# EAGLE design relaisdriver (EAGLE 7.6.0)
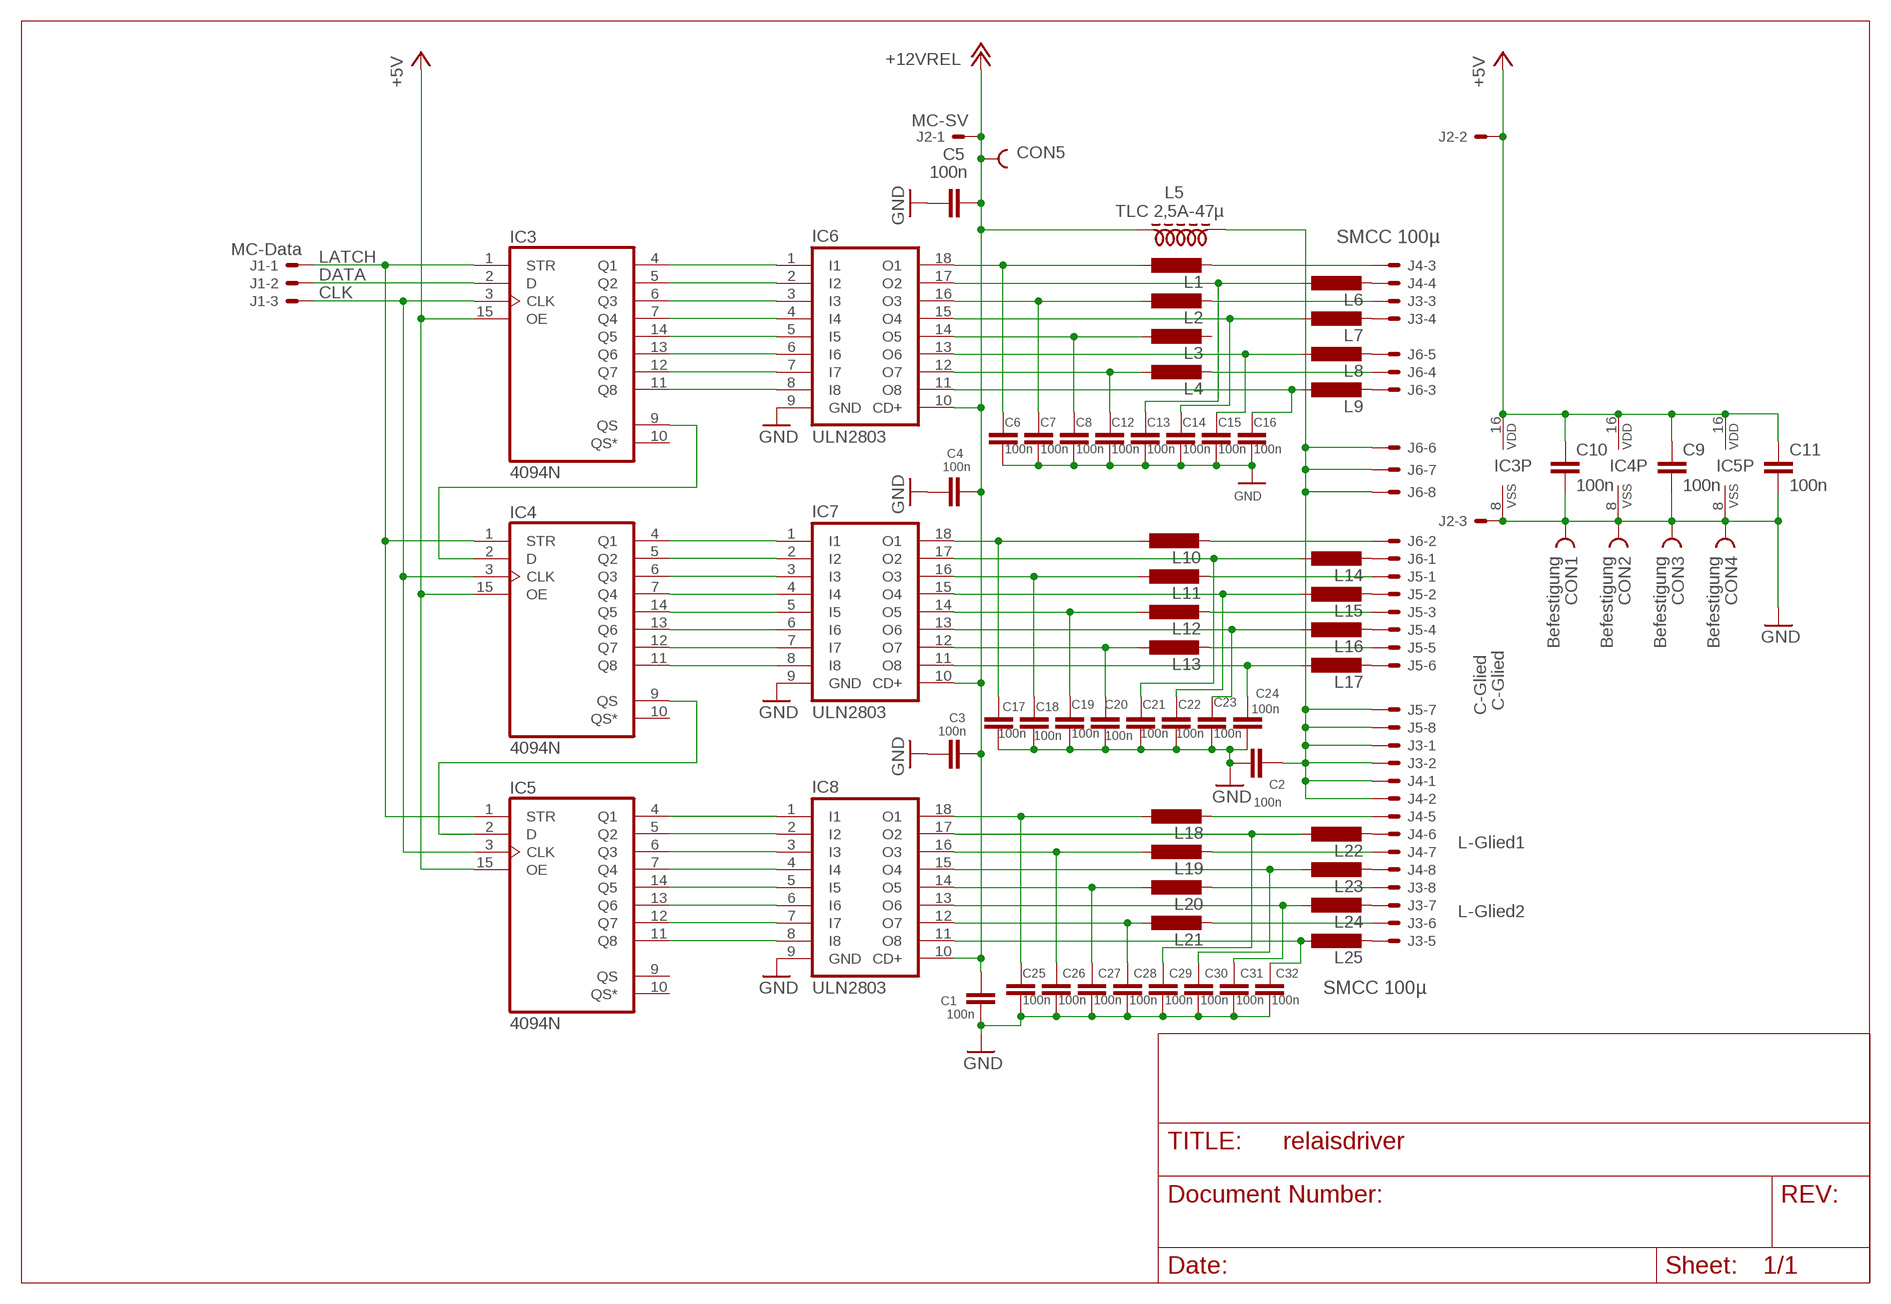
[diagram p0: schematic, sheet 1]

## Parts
C1  100n  C-EUC0805  [C0805]
C2  100n  C-EUC0805  [C0805]
C3  100n  C-EUC0805  [C0805]
C4  100n  C-EUC0805  [C0805]
C5  100n  C-EUC0805  [C0805]
C6  100n  C-EUC0805  [C0805]
C7  100n  C-EUC0805  [C0805]
C8  100n  C-EUC0805  [C0805]
C9  100n  C-EUC0805  [C0805]
C10  100n  C-EUC0805  [C0805]
C11  100n  C-EUC0805  [C0805]
C12  100n  C-EUC0805  [C0805]
C13  100n  C-EUC0805  [C0805]
C14  100n  C-EUC0805  [C0805]
C15  100n  C-EUC0805  [C0805]
C16  100n  C-EUC0805  [C0805]
C17  100n  C-EUC0805  [C0805]
C18  100n  C-EUC0805  [C0805]
C19  100n  C-EUC0805  [C0805]
C20  100n  C-EUC0805  [C0805]
C21  100n  C-EUC0805  [C0805]
C22  100n  C-EUC0805  [C0805]
C23  100n  C-EUC0805  [C0805]
C24  100n  C-EUC0805  [C0805]
C25  100n  C-EUC0805  [C0805]
C26  100n  C-EUC0805  [C0805]
C27  100n  C-EUC0805  [C0805]
C28  100n  C-EUC0805  [C0805]
C29  100n  C-EUC0805  [C0805]
C30  100n  C-EUC0805  [C0805]
C31  100n  C-EUC0805  [C0805]
C32  100n  C-EUC0805  [C0805]
CON1  Befestigung  PIN2_53MM  [HOLE3]
CON2  Befestigung  PIN2_53MM  [HOLE3]
CON3  Befestigung  PIN2_53MM  [HOLE3]
CON4  Befestigung  PIN2_53MM  [HOLE3]
CON5  PIN1_75OV  [PIN_1,75OV]
IC3  4094N  [DIL16]
IC4  4094N  [DIL16]
IC5  4094N  [DIL16]
IC6  ULN2803  ULN2803A  [DIL18]
IC7  ULN2803  ULN2803A  [DIL18]
IC8  ULN2803  ULN2803A  [DIL18]
J1  MC-Data  22-27-2031-03  [6410-03]
J2  MC-SV  22-27-2031-03  [6410-03]
J3  L-Glied2  22-27-2081-08  [6410-08]
J4  L-Glied1  22-27-2081-08  [6410-08]
J5  C-Glied  22-27-2081-08  [6410-08]
J6  C-Glied  22-27-2081-08  [6410-08]
L1  L-EU0207/10  [0207/10]
L2  L-EU0207/10  [0207/10]
L3  L-EU0207/10  [0207/10]
L4  L-EU0207/10  [0207/10]
L5  TLC 2,5A-47µ  Z28/70CW  [Z28/7]
L6  L-EU0207/10  [0207/10]
L7  L-EU0207/10  [0207/10]
L8  L-EU0207/10  [0207/10]
L9  L-EU0207/10  [0207/10]
L10  L-EU0207/10  [0207/10]
L11  L-EU0207/10  [0207/10]
L12  L-EU0207/10  [0207/10]
L13  L-EU0207/10  [0207/10]
L14  L-EU0207/10  [0207/10]
L15  L-EU0207/10  [0207/10]
L16  L-EU0207/10  [0207/10]
L17  L-EU0207/10  [0207/10]
L18  L-EU0207/10  [0207/10]
L19  L-EU0207/10  [0207/10]
L20  L-EU0207/10  [0207/10]
L21  L-EU0207/10  [0207/10]
L22  L-EU0207/10  [0207/10]
L23  L-EU0207/10  [0207/10]
L24  L-EU0207/10  [0207/10]
L25  L-EU0207/10  [0207/10]

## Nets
+5V: C9.1 C10.1 C11.1 IC3.15(OE) IC3.16(VDD) IC4.15(OE) IC4.16(VDD) IC5.15(OE) IC5.16(VDD) J2.2
+12VREL: C1.1 C3.1 C4.1 C5.1 CON5.1 IC6.10(CD+) IC7.10(CD+) IC8.10(CD+) J2.1 L5.1 ; supply symbol labelled +12V
CLK: IC3.3(CLK) IC4.3(CLK) IC5.3(CLK) J1.3
DATA: IC3.2(D) J1.2
GND: C1.2 C2.2 C3.2 C4.2 C5.2 C6.2 C7.2 C8.2 C9.2 C10.2 C11.2 C12.2 C13.2 C14.2 C15.2 C16.2 C17.2 C18.2 C19.2 C20.2 C21.2 C22.2 C23.2 C24.2 C25.2 C26.2 C27.2 C28.2 C29.2 C30.2 C31.2 C32.2 CON1.1 CON2.1 CON3.1 CON4.1 IC3.8(VSS) IC4.8(VSS) IC5.8(VSS) IC6.9(GND) IC7.9(GND) IC8.9(GND) J2.3
LATCH: IC3.1(STR) IC4.1(STR) IC5.1(STR) J1.1
N$1: C6.1 IC6.18(O1) L1.1
N$2: C7.1 IC6.16(O3) L2.1
N$3: IC4.7(Q4) IC7.4(I4)
N$4: IC4.14(Q5) IC7.5(I5)
N$5: IC4.13(Q6) IC7.6(I6)
N$6: C8.1 IC6.14(O5) L3.1
N$7: C12.1 IC6.12(O7) L4.1
N$8: C16.1 IC6.11(O8) L9.1
N$9: IC3.4(Q1) IC6.1(I1)
N$10: C15.1 IC6.13(O6) L8.1
N$11: C14.1 IC6.15(O4) L7.1
N$12: IC4.12(Q7) IC7.7(I7)
N$13: C13.1 IC6.17(O2) L6.1
N$14: IC4.11(Q8) IC7.8(I8)
N$15: J4.4 L6.2
N$16: J3.5 L25.2
N$17: J3.6 L21.2
N$18: J6.4 L4.2
N$19: J6.2 L10.2
N$20: J5.1 L11.2
N$21: IC3.5(Q2) IC6.2(I2)
N$22: IC3.6(Q3) IC6.3(I3)
N$23: IC3.9(QS) IC4.2(D)
N$24: IC4.9(QS) IC5.2(D)
N$25: IC3.7(Q4) IC6.4(I4)
N$26: IC3.14(Q5) IC6.5(I5)
N$27: IC3.13(Q6) IC6.6(I6)
N$28: IC3.12(Q7) IC6.7(I7)
N$29: IC3.11(Q8) IC6.8(I8)
N$30: IC4.4(Q1) IC7.1(I1)
N$31: IC4.5(Q2) IC7.2(I2)
N$32: IC4.6(Q3) IC7.3(I3)
N$33: J5.3 L12.2
N$34: J5.5 L13.2
N$35: J4.8 L23.2
N$36: C17.1 IC7.18(O1) L10.1
N$37: C18.1 IC7.16(O3) L11.1
N$38: IC5.4(Q1) IC8.1(I1)
N$39: IC5.5(Q2) IC8.2(I2)
N$40: IC5.6(Q3) IC8.3(I3)
N$41: IC5.7(Q4) IC8.4(I4)
N$42: IC5.14(Q5) IC8.5(I5)
N$43: IC5.13(Q6) IC8.6(I6)
N$44: IC5.12(Q7) IC8.7(I7)
N$45: IC5.11(Q8) IC8.8(I8)
N$46: C19.1 IC7.14(O5) L12.1
N$47: C20.1 IC7.12(O7) L13.1
N$48: C24.1 IC7.11(O8) L17.1
N$49: C23.1 IC7.13(O6) L16.1
N$50: C22.1 IC7.15(O4) L15.1
N$51: C21.1 IC7.17(O2) L14.1
N$52: C2.1 J3.1 J3.2 J4.1 J4.2 J5.7 J5.8 J6.6 J6.7 J6.8 L5.2
N$53: J5.6 L17.2
N$54: J5.4 L16.2
N$55: J5.2 L15.2
N$56: J6.1 L14.2
N$57: J6.3 L9.2
N$58: J6.5 L8.2
N$59: J3.7 L24.2
N$60: C25.1 IC8.18(O1) L18.1
N$61: C26.1 IC8.16(O3) L19.1
N$62: C27.1 IC8.14(O5) L20.1
N$63: C28.1 IC8.12(O7) L21.1
N$64: C32.1 IC8.11(O8) L25.1
N$65: C31.1 IC8.13(O6) L24.1
N$66: C30.1 IC8.15(O4) L23.1
N$67: C29.1 IC8.17(O2) L22.1
N$68: J4.5 L18.2
N$69: J4.6 L22.2
N$70: J4.7 L19.2
N$71: J4.3 L1.2
N$72: J3.8 L20.2
N$73: J3.4 L7.2
N$74: J3.3 L2.2
Unconnected: IC3.10(QS*) IC4.10(QS*) IC5.9(QS) IC5.10(QS*) L3.2

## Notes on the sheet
- SMCC 100µ
- SMCC 100µ

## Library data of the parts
C1-C32 = rcl:C-EU: CAPACITOR, European symbol
CON1-CON4 = lindenau:PIN2_5
CON5 = lindenau:PIN1_75
IC3-IC5 = 40xx:4094: 8-stage SHIFT/STORE REGISTER, tri-state
IC6-IC8 = uln-udn:ULN2803A: DRIVER ARRAY
J1 J2 = con-molex:22-?-03: CONNECTOR wire to board 2.54 mm (.1 inch) pitch header; OC_FARNELL: unknown; OC_NEWARK: unknown
J3-J6 = con-molex:22-?-08: CONNECTOR wire to board 2.54 mm (.1 inch) pitch header; OC_FARNELL: unknown; OC_NEWARK: unknown
L1-L4 L6-L25 = rcl:L-EU: INDUCTOR, European symbol
L5 = inductor-neosid:Z?CW: CHOKE; OC_FARNELL: unknown; OC_NEWARK: unknown

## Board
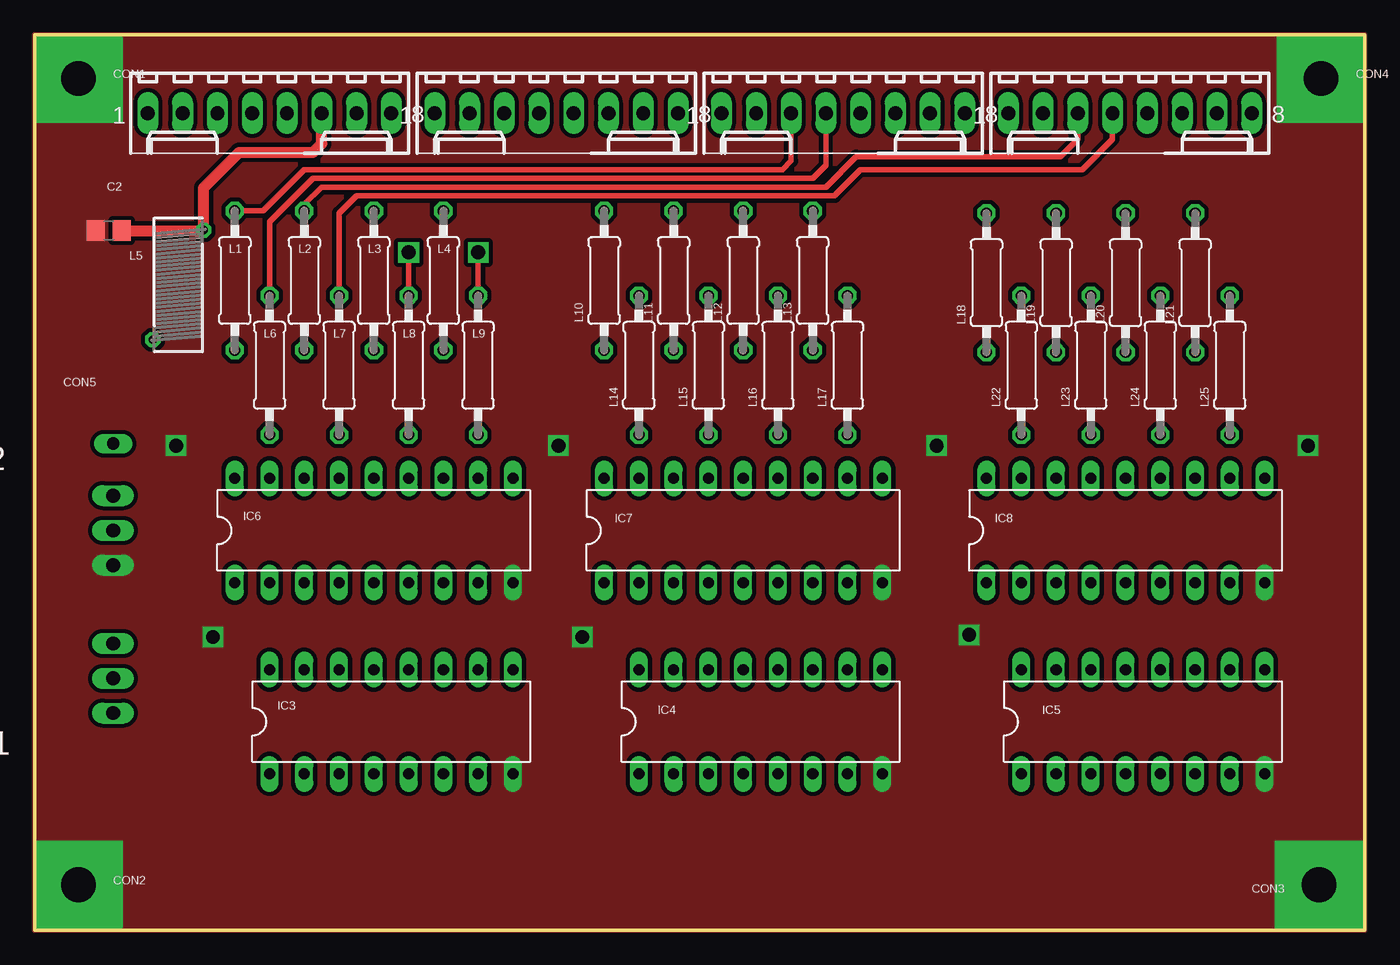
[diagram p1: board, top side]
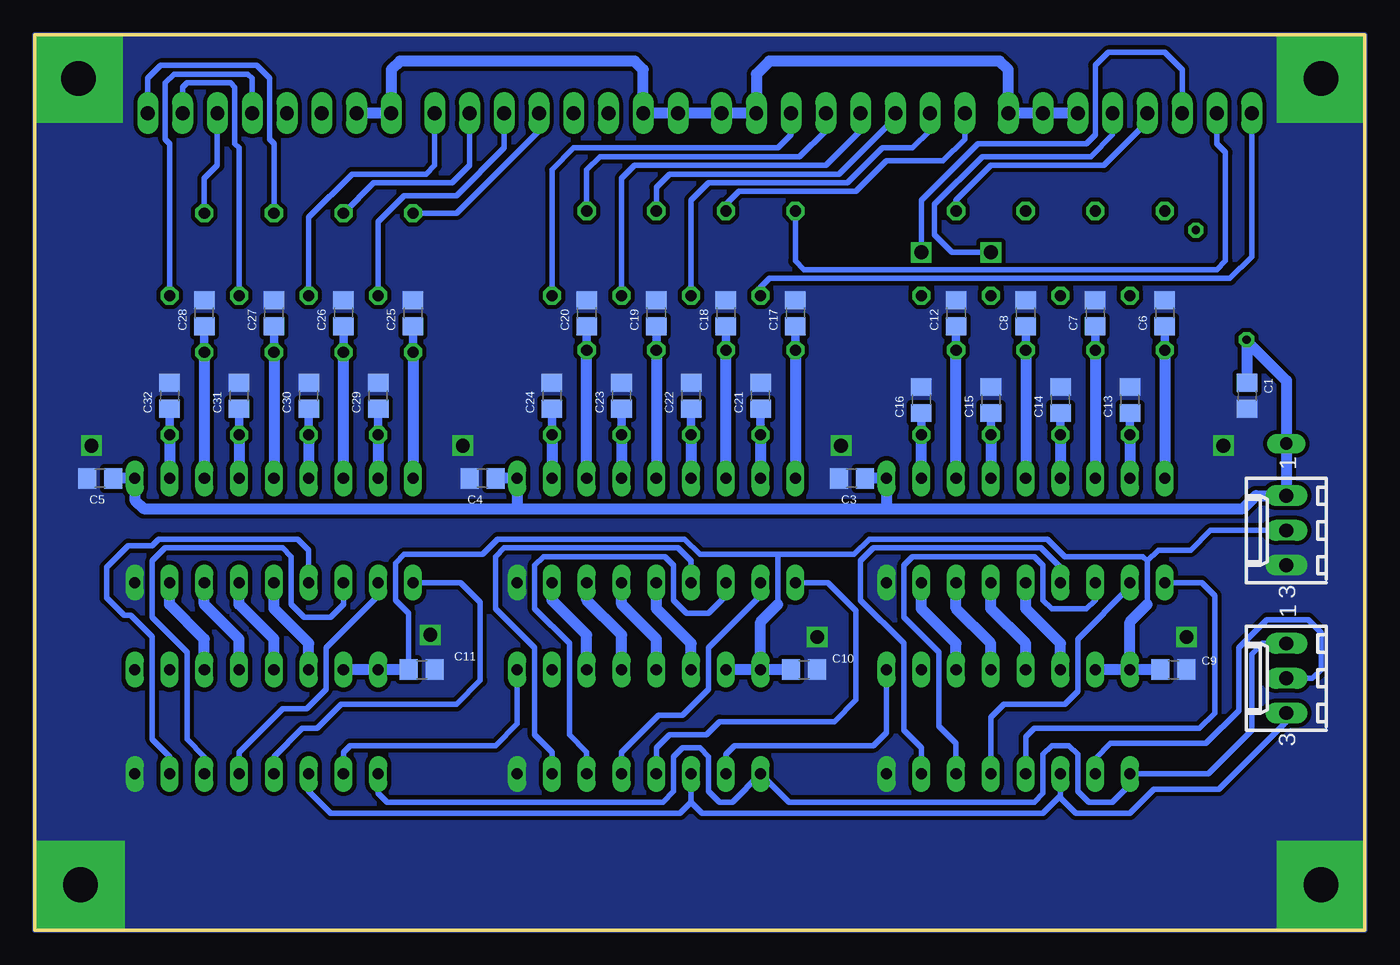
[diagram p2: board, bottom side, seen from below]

Size 97.16 x 65.41 mm. Coordinates in mm from the lower left corner, seen from the top.
Outline: 0,65.41 97.16,65.41 97.16,0 0,0 0,65.41
Copper layers (1*16): Top 0.035mm / dielectric 1.5mm / Bottom 0.035mm
Design rules "default *": minimum track width 10mil, minimum drill 24mil, track to track 8mil, track to pad 8mil, pad to pad 8mil, via to via 8mil, smd to smd 8mil, copper to edge 0mil, drill to drill 8mil, minimum pad ring 10mil, minimum via ring 8mil, stop-mask expansion 4mil, vias tented up to drill 0mil, thermal gap 10mil

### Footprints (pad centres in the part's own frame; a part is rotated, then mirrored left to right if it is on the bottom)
C0805 = smd 1.3 x 1.5: 1 -0.95,0; 2 0.95,0
HOLE3 = drill 2.54 pad 6.452 square: 1 0,0
PIN_1,75OV = drill 0.9 pad 1.397 long: 1 0,0
DIL16 = drill 0.813 long: 1 -8.89,-3.81; 2 -6.35,-3.81; 3 -3.81,-3.81; 4 -1.27,-3.81; 5 1.27,-3.81; 6 3.81,-3.81; 7 6.35,-3.81; 8 8.89,-3.81; 9 8.89,3.81; 10 6.35,3.81; 11 3.81,3.81; 12 1.27,3.81; 13 -1.27,3.81; 14 -3.81,3.81; 15 -6.35,3.81; 16 -8.89,3.81
DIL18 = drill 0.813 long: 1 -10.16,-3.81; 2 -7.62,-3.81; 3 -5.08,-3.81; 4 -2.54,-3.81; 5 0,-3.81; 6 2.54,-3.81; 7 5.08,-3.81; 8 7.62,-3.81; 9 10.16,-3.81; 10 10.16,3.81; 11 7.62,3.81; 12 5.08,3.81; 13 2.54,3.81; 14 0,3.81; 15 -2.54,3.81; 16 -5.08,3.81; 17 -7.62,3.81; 18 -10.16,3.81
6410-03 = drill 1.016 long: 1 2.54,0; 2 0,0; 3 -2.54,0
6410-08 = drill 1.016 long: 1 8.89,0; 2 6.35,0; 3 3.81,0; 4 1.27,0; 5 -1.27,0; 6 -3.81,0; 7 -6.35,0; 8 -8.89,0
0207/10 = drill 0.813 octagon: 1 -5.08,0; 2 5.08,0
Z28/7 = drill 0.6 octagon: 1 4,-1.85; 2 -4,1.85

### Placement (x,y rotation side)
C1  8.57,39.05 270 bottom
C2  5.4,51.12 180 top
C3  37.47,33.02 180 bottom
C4  64.45,33.02 180 bottom
C5  92.39,33.02 180 bottom
C6  14.61,45.09 90 bottom
C7  19.68,45.09 90 bottom
C8  24.77,45.09 90 bottom
C9  13.97,19.05 0 bottom
C10  40.96,19.05 0 bottom
C11  68.9,19.05 0 bottom
C12  29.84,45.09 90 bottom
C13  17.14,38.73 90 bottom
C14  22.23,38.73 90 bottom
C15  27.3,38.73 90 bottom
C16  32.38,38.73 90 bottom
C17  41.59,45.09 90 bottom
C18  46.67,45.09 90 bottom
C19  51.75,45.09 90 bottom
C20  56.83,45.09 90 bottom
C21  44.13,39.05 90 bottom
C22  49.21,39.05 90 bottom
C23  54.29,39.05 90 bottom
C24  59.37,39.05 90 bottom
C25  69.53,45.09 90 bottom
C26  74.61,45.09 90 bottom
C27  79.69,45.09 90 bottom
C28  84.77,45.09 90 bottom
C29  72.07,39.05 90 bottom
C30  77.15,39.05 90 bottom
C31  82.23,39.05 90 bottom
C32  87.31,39.05 90 bottom
CON1  3.17,62.23 0 top
CON2  3.17,3.33 0 top
CON3  93.82,3.33 180 top
CON4  93.98,62.23 0 top
CON5  5.71,35.56 180 top
IC3  26.04,15.24 0 top
IC4  53.02,15.24 0 top
IC5  80.96,15.24 0 top
IC6  24.77,29.21 0 top
IC7  51.75,29.21 0 top
IC8  79.69,29.21 0 top
J1  5.71,18.41 90 bottom
J2  5.71,29.21 90 bottom
J3  80.01,59.69 180 top
J4  59.05,59.69 180 top
J5  38.1,59.69 180 top
J6  17.14,59.69 180 top
L1  14.61,47.47 90 top
L2  19.68,47.47 90 top
L3  24.77,47.47 90 top
L4  29.84,47.47 90 top
L5  10.48,47.15 270 top
L6  17.14,41.27 90 top
L7  22.23,41.27 90 top
L8  27.3,41.27 90 top
L9  32.38,41.27 90 top
L10  41.59,47.47 90 top
L11  46.67,47.47 90 top
L12  51.75,47.47 90 top
L13  56.83,47.47 90 top
L14  44.13,41.27 90 top
L15  49.21,41.27 90 top
L16  54.29,41.27 90 top
L17  59.37,41.27 90 top
L18  69.53,47.31 90 top
L19  74.61,47.31 90 top
L20  79.69,47.31 90 top
L21  84.77,47.31 90 top
L22  72.07,41.27 90 top
L23  77.15,41.27 90 top
L24  82.23,41.27 90 top
L25  87.31,41.27 90 top

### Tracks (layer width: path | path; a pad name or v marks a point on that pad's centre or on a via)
+5V
  Bottom 0.406: 15.88,23.81 15.88,26.99 | 15.88,26.99 15.08,27.78 12.7,27.78 11.27,29.21 J2.2 | C11.1 69.85,23.18 70.8,24.13 70.8,26.83 70.17,27.46 64.45,27.46 63.34,28.57 49.69,28.57 48.58,27.46 42.86,27.46 | 42.86,27.46 37.31,27.46 36.2,28.57 23.18,28.57 21.91,27.3 16.19,27.3 15.88,26.99 | 42.86,23.81 42.86,27.46
  Bottom 0.813: C11.1 IC5.16 IC5.15 | C10.1 IC4.16 | C9.1 IC3.16 | IC3.16 IC3.15 | IC4.16 IC4.15 | IC4.16 44.13,22.54 42.86,23.81 | IC3.16 17.14,22.54 15.88,23.81
+12VREL
  Bottom 0.813: 61.91,30.8 89.22,30.8 89.85,31.43 IC8.10 C5.1 | 61.91,30.8 34.92,30.8 | 34.92,30.8 8.89,30.8 7.94,31.75 J2.1 CON5.1 5.71,40.16 8.63,43.08 L5.1 8.57,43.09 C1.1 | 34.92,30.8 IC6.10 C3.1 | 61.91,30.8 IC7.10 C4.1
CLK
  Bottom 0.406: 49.21,9.37 48.42,8.57 23.5,8.57 22.23,9.84 IC3.3 22.23,9.68 21.11,8.57 17.14,8.57 15.4,10.32 10.64,10.32 5.71,15.24 J1.3 | IC4.3 49.21,9.37 | 49.21,9.37 50.01,8.57 75.56,8.57 77.15,10.16 IC5.3
DATA
  Bottom 0.406: IC3.2 19.68,12.54 18.57,13.65 11.59,13.65 9.21,16.03 9.21,20.64 7.14,22.7 4.13,22.7 3.17,21.75 3.17,19.05 3.81,18.41 J1.2
GND  (via drill 1)
  other vias: 40.01,21.43 68.26,21.59 13.02,21.43 10.32,35.4 38.26,35.4 65.88,35.4 93.03,35.4
  pour Bottom (isolate 0.305, no thermals): 0,65.41 0,0 97.16,0 97.16,65.41
  pour Top (isolate 0.305, no thermals): 0,65.41 0,0 97.16,0 97.16,65.41
LATCH
  Bottom 0.406: IC5.1 72.07,10 71.44,9.37 51.28,9.37 50.48,10.16 50.48,12.7 49.85,13.34 48.58,13.34 47.94,12.7 47.94,10.16 47.15,9.37 46.2,9.37 IC4.1 42.07,9.37 24.13,9.37 23.5,10 23.5,12.86 22.86,13.49 21.59,13.49 20.95,12.86 20.95,10.16 20.16,9.37 18.41,9.37 17.14,10.64 IC3.1 11.43,11.43 8.26,14.61 8.26,20.16 7.46,20.95 J1.1
N$1
  Bottom 0.61: C6.1 L1.1
  Bottom 0.813: L1.1 IC6.18
N$2
  Bottom 0.61: C7.1 L2.1
  Bottom 0.813: L2.1 IC6.16
N$3
  Bottom 0.406: IC4.7 59.37,13.02 60.64,14.29 60.64,20.64 63.5,23.5 63.5,27.3 62.87,27.94 50.16,27.94 49.21,26.99 IC7.4
N$4
  Bottom 0.813: IC4.14 49.21,20.95 51.75,23.5 IC7.5
N$5
  Bottom 0.813: IC4.13 51.75,21.27 54.29,23.81 IC7.6
N$6
  Bottom 0.61: C8.1 L3.1
  Bottom 0.813: L3.1 IC6.14
N$7
  Bottom 0.61: C12.1 L4.1
  Bottom 0.813: IC6.12 L4.1
N$8
  Bottom 0.61: C16.1 L9.1
  Bottom 0.813: IC6.11 L9.1
N$9
  Bottom 0.406: IC3.4 24.77,14.13 24.13,14.76 12.06,14.76 10.95,15.88 10.95,24.45 11.91,25.4 IC6.1
N$10
  Bottom 0.61: C15.1 L8.1
  Bottom 0.813: L8.1 IC6.13
N$11
  Bottom 0.61: C14.1 L7.1
  Bottom 0.813: L7.1 IC6.15
N$12
  Bottom 0.813: IC4.12 54.29,21.59 56.83,24.13 IC7.7
N$13
  Bottom 0.61: C13.1 L6.1
  Bottom 0.813: L6.1 IC6.17
N$14
  Bottom 0.813: IC4.11 56.83,21.59 59.37,24.13 IC7.8
N$15
  Top 0.406: L6.2 17.14,51.75 20.32,54.93 56.83,54.93 57.78,55.88 J4.4
N$16
  Bottom 0.406: L25.2 87.31,57.47 87.63,57.78 87.63,61.91 87,62.55 81.6,62.55 81.28,62.23 J3.5
N$17
  Bottom 0.406: J3.6 83.82,55.88 84.77,54.93 L21.2
N$18
  Bottom 0.406: J6.4 15.88,59.05 19.05,55.88 27.3,55.88 29.84,53.34 L4.2
N$19
  Bottom 0.406: L10.2 41.59,48.9 40.96,48.26 10.79,48.26 10.16,48.9 10.16,56.83 10.79,57.47 J6.2
N$20
  Bottom 0.406: J5.1 29.21,57.78 30.8,56.2 34.92,56.2 37.15,53.98 45.72,53.98 46.67,53.02 L11.2
N$21
  Bottom 0.406: IC6.2 17.14,25.08 20.95,21.27 20.95,17.46 21.91,16.51 26.35,16.51 27.3,15.56 IC3.5
N$22
  Bottom 0.406: IC3.6 29.84,13.65 31.11,14.92 31.11,20.32 33.66,22.86 33.66,26.67 33.02,27.3 24.13,27.3 23.5,26.67 23.5,24.13 22.86,23.5 20.32,23.5 19.68,24.13 IC6.3
N$23
  Bottom 0.406: IC4.2 46.67,12.86 46.04,13.49 35.88,13.49 34.92,14.45 IC3.9
N$24
  Bottom 0.406: IC4.9 61.91,15.08 63.5,13.49 74.14,13.49 74.61,13.02 IC5.2
N$25
  Bottom 0.406: IC3.7 32.38,13.34 33.66,14.61 33.66,20.95 36.83,24.13 36.83,26.99 35.88,27.94 23.65,27.94 22.23,26.51 IC6.4
N$26
  Bottom 0.813: IC6.5 24.77,23.5 22.23,20.95 IC3.14
N$27
  Bottom 0.813: IC6.6 27.3,23.5 24.77,20.95 IC3.13
N$28
  Bottom 0.813: IC6.7 29.84,23.5 27.3,20.95 IC3.12
N$29
  Bottom 0.813: IC6.8 32.38,23.5 29.84,20.95 IC3.11
N$30
  Bottom 0.406: IC4.4 51.75,13.34 50.8,14.29 48.1,14.29 47.15,15.24 38.73,15.24 37.15,16.83 37.15,23.34 39.21,25.4 IC7.1
N$31
  Bottom 0.406: IC7.2 44.13,24.45 47.94,20.64 47.94,17.62 49.85,15.72 51.59,15.72 54.29,13.02 IC4.5
N$32
  Bottom 0.406: IC7.3 46.67,24.45 47.94,23.18 49.53,23.18 50.48,24.13 50.48,26.67 51.12,27.3 60.01,27.3 60.64,26.67 60.64,23.5 58.1,20.95 58.1,14.29 56.83,13.02 IC4.6
N$33
  Bottom 0.406: J5.3 34.29,59.37 38.42,55.24 50.8,55.24 51.75,54.29 L12.2
N$34
  Bottom 0.406: J5.5 39.37,58.42 41.27,56.52 55.88,56.52 56.83,55.56 L13.2
N$35
  Bottom 0.406: J4.8 67.94,55.88 68.58,55.24 73.98,55.24 77.15,52.07 L23.2
N$36
  Bottom 0.61: C17.1 L10.1
  Bottom 0.813: L10.1 IC7.18
N$37
  Bottom 0.61: C18.1 L11.1
  Bottom 0.813: IC7.16 L11.1
N$38
  Bottom 0.406: IC5.4 79.69,12.7 77.63,14.76 76.52,14.76 74.77,16.51 66.36,16.51 64.61,18.26 64.61,23.97 66.04,25.4 IC8.1
N$39
  Bottom 0.406: IC8.2 72.07,24.45 75.88,20.64 75.88,17.62 77.31,16.19 79.06,16.19 82.23,13.02 IC5.5
N$40
  Bottom 0.406: IC8.3 74.61,23.81 75.56,22.86 77.47,22.86 78.42,23.81 78.42,27.3 79.06,27.94 87.63,27.94 88.58,26.99 88.58,22.86 86.04,20.32 86.04,13.97 84.77,12.7 IC5.6
N$41
  Bottom 0.406: IC5.7 87.31,12.7 88.58,13.97 88.58,21.43 90.17,23.02 90.65,23.02 91.92,24.29 91.92,26.51 90.33,28.1 88.58,28.1 88.11,28.57 77.95,28.57 77.15,27.78 IC8.4
N$42
  Bottom 0.813: IC5.14 77.15,20.95 79.69,23.5 IC8.5
N$43
  Bottom 0.813: IC5.13 79.69,21.27 82.23,23.81 IC8.6
N$44
  Bottom 0.813: IC5.12 82.23,21.27 84.77,23.81 IC8.7
N$45
  Bottom 0.813: IC5.11 84.77,21.27 87.31,23.81 IC8.8
N$46
  Bottom 0.61: C19.1 L12.1
  Bottom 0.813: L12.1 IC7.14
N$47
  Bottom 0.61: C20.1 L13.1
  Bottom 0.813: IC7.12 L13.1
N$48
  Bottom 0.61: C24.1 L17.1
  Bottom 0.813: L17.1 IC7.11
N$49
  Bottom 0.61: C23.1 L16.1
  Bottom 0.813: L16.1 IC7.13
N$50
  Bottom 0.61: C22.1 L15.1
  Bottom 0.813: L15.1 IC7.15
N$51
  Bottom 0.61: C21.1 L14.1
  Bottom 0.813: L14.1 IC7.17
N$52
  Top 0.813: J6.6 20.95,57.47 20.32,56.83 14.92,56.83 12.33,54.24 L5.2 12.3,51.12 C2.1
  Bottom 0.813: J6.6 J6.7 J6.8 26.04,62.87 26.67,63.5 43.5,63.5 44.45,62.55 J5.7 J5.8 J4.1 J4.2 52.7,62.87 53.34,63.5 70.48,63.5 71.12,62.87 J3.1 J3.2
N$53
  Bottom 0.406: J5.6 41.91,58.1 42.86,57.15 57.78,57.15 59.37,55.56 L17.2
N$54
  Bottom 0.406: J5.4 36.83,58.42 39.37,55.88 53.34,55.88 54.29,54.93 L16.2
N$55
  Bottom 0.406: J5.2 31.75,58.42 33.02,57.15 35.24,57.15 37.78,54.61 47.94,54.61 49.21,53.34 L15.2
N$56
  Bottom 0.406: J6.1 8.26,49.21 9.84,47.62 43.5,47.62 44.13,46.99 L14.2
N$57  (via drill 1)
  Top 0.406: v32.38,49.53 L9.2
  Bottom 0.406: J6.3 13.34,62.87 14.61,64.14 18.73,64.14 19.68,63.18 19.68,58.1 20.32,57.47 28.26,57.47 32.38,53.34 v32.38,49.53
N$58  (via drill 1)
  Top 0.406: v27.3,49.53 L8.2
  Bottom 0.406: J6.5 18.41,58.1 20,56.52 27.94,56.52 31.43,53.02 31.43,50.8 30.16,49.53 v27.3,49.53
N$59
  Bottom 0.406: L24.2 82.23,57.15 82.55,57.47 82.55,61.59 82.87,61.91 86.04,61.91 86.36,61.59 J3.7
N$60
  Bottom 0.61: C25.1 L18.1
  Bottom 0.813: L18.1 IC8.18
N$61
  Bottom 0.61: C26.1 L19.1
  Bottom 0.813: IC8.16 L19.1
N$62
  Bottom 0.61: C27.1 L20.1
  Bottom 0.813: L20.1 IC8.14
N$63
  Bottom 0.61: C28.1 L21.1
  Bottom 0.813: L21.1 IC8.12
N$64
  Bottom 0.61: C32.1 L25.1
  Bottom 0.813: L25.1 IC8.11
N$65
  Bottom 0.61: C31.1 L24.1
  Bottom 0.813: L24.1 IC8.13
N$66
  Bottom 0.61: C30.1 L23.1
  Bottom 0.813: L23.1 IC8.15
N$67
  Bottom 0.61: C29.1 L22.1
  Bottom 0.813: L22.1 IC8.17
N$68
  Bottom 0.406: J4.5 60.33,58.42 66.36,52.39 L18.2
N$69
  Bottom 0.406: J4.6 62.87,57.15 66.36,53.66 70.17,53.66 72.07,51.75 L22.2
N$70
  Bottom 0.406: J4.7 65.41,55.88 66.67,54.61 72.39,54.61 L19.2
N$71
  Top 0.406: L1.2 16.67,52.55 19.68,55.56 54.61,55.56 55.24,56.2 J4.3
N$72
  Bottom 0.406: L20.2 79.69,57.47 80.01,57.78 80.01,62.23 80.96,63.18 87.95,63.18 88.9,62.23 J3.8
N$73
  Top 0.406: L7.2 22.23,52.39 23.5,53.66 58.42,53.66 60.33,55.56 76.52,55.56 78.74,57.78 J3.4
N$74
  Top 0.406: L2.2 19.68,53.02 20.95,54.29 57.78,54.29 60.01,56.52 74.93,56.52 76.2,57.78 J3.3

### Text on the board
Document: KC7 | KC8 | KC9 | KC10 | KC11 | KC6 | KC5 | KC4 | KC3 | KC2 | KC1 | KLC4 | KLC3 | KL8 | KL7 | KL6 | KL5 | KLC2 | KLC1 | KL1 | KL2 | KL3 | KL4
tDocu: 12V R | 5V | GND | Latch | Cdata | CLK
